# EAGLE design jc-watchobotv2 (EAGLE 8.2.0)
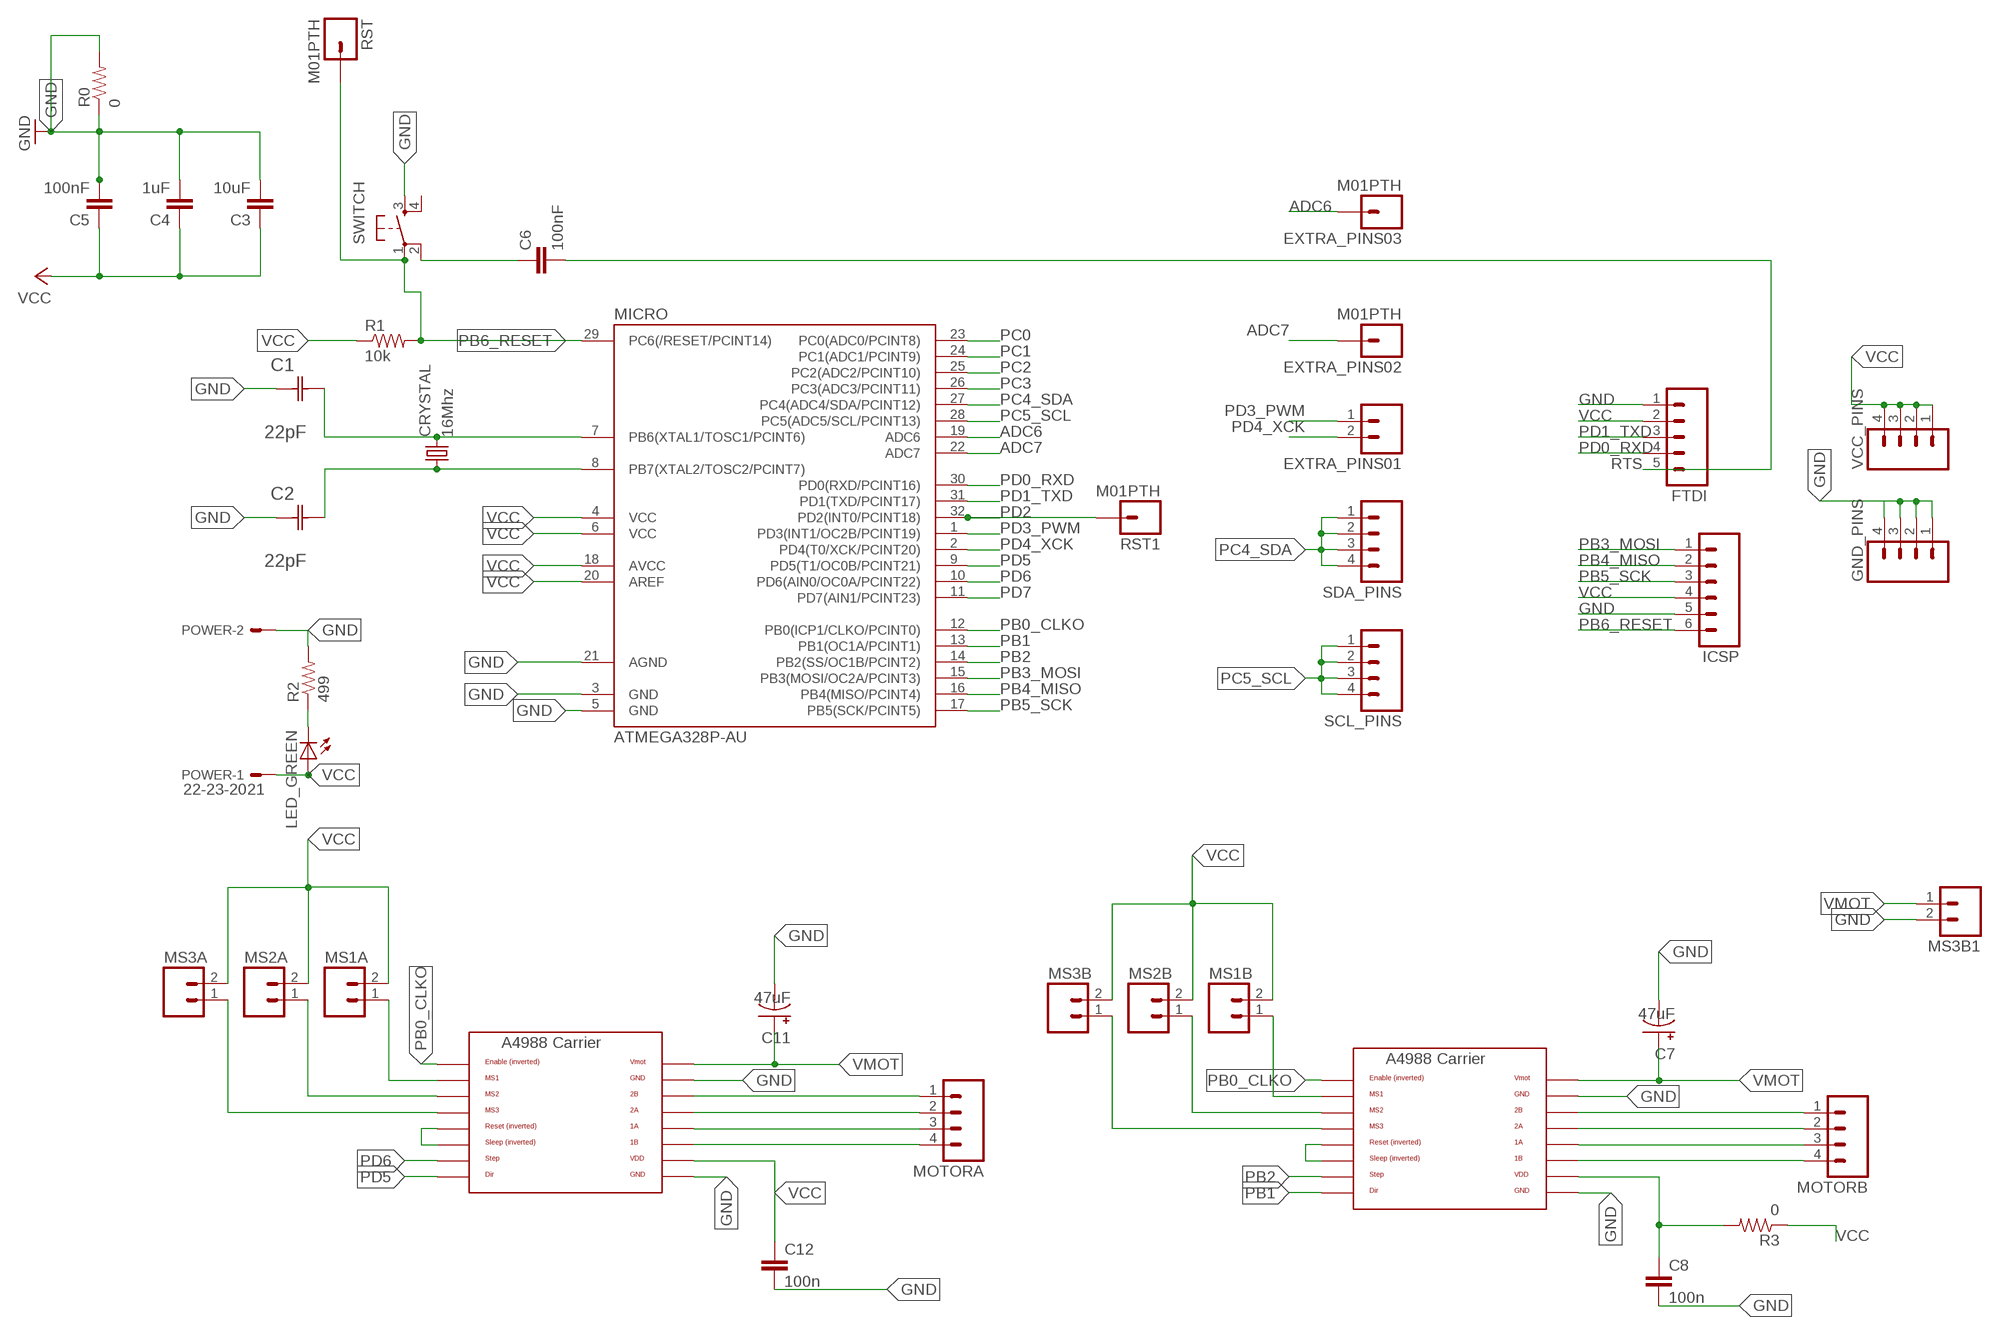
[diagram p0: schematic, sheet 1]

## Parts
C1  22pF  0612ZC225MAT2A  [CAPC3216X178N]
C2  22pF  0612ZC225MAT2A  [CAPC3216X178N]
C3  10uF  CAP1206  [1206]
C4  1uF  CAP1206  [1206]
C5  100nF  CAP1206  [1206]
C6  100nF  CAP1206  [1206]
C7  47uF  MCGPR50V107M8X11  [MCGPR50V107M8X11]
C8  100n  CAP1206  [1206]
C11  47uF  MCGPR50V107M8X11  [MCGPR50V107M8X11]
C12  100n  CAP1206  [1206]
CRYSTAL  16Mhz  CSM-7X-DU  [CSM-7X-DU]
EXTRA_PINS01  M02  [02P]
EXTRA_PINS02  M01PTH  [1X01]
EXTRA_PINS03  M01PTH  [1X01]
FTDI  M05  [05P]
GND_PINS  M04  [04P]
ICSP  M06  [06P]
LED_GREEN  LED1206  [1206]
MICRO  ATMEGA328P-AU  ATMEGA48/88/168-AU  [TQFP32-08]
MOTORA  M04  [04P]
MOTORA_CARRIER  A4988BREAKOUT  [A4988BREAKOUT]
MOTORB  M04  [04P]
MOTORB_CARRIER  A4988BREAKOUT  [A4988BREAKOUT]
MS1A  M02  [02P]
MS1B  M02  [02P]
MS2A  M02  [02P]
MS2B  M02  [02P]
MS3A  M02  [02P]
MS3B  M02  [02P]
MS3B1  M02  [02P]
POWER  22-23-2021  [22-23-2021]
R0  0  RESISTOR1206  [1206]
R1  10k  RESISTOR1206  [1206]
R2  499  RESISTOR1206  [1206]
R3  0  RESISTOR1206  [1206]
RST  M01PTH  [1X01]
RST1  M01PTH  [1X01]
SCL_PINS  M04  [04P]
SDA_PINS  M04  [04P]
SWITCH  6MM_SWITCH6MM_SWITCH  [6MM_SWITCH]
VCC_PINS  M04  [04P]

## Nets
ADC6: EXTRA_PINS03.1 MICRO.19(ADC6)
ADC7: EXTRA_PINS02.1 MICRO.22(ADC7)
GND: C1.1(C1) C2.1(C1) C3.2 C4.2 C5.2 C7.- C8.2 C11.- C12.2 FTDI.1 GND_PINS.1 GND_PINS.2 GND_PINS.3 GND_PINS.4 ICSP.5 MICRO.3(GND) MICRO.5(GND) MICRO.21(AGND) MOTORA_CARRIER.GND MOTORA_CARRIER.GND@0(GND) MOTORB_CARRIER.GND MOTORB_CARRIER.GND@0(GND) MS3B1.2 POWER.2 R0.1 R0.2 R2.2 SWITCH.3(S)
N$1: MOTORB_CARRIER.MS1 MS1B.1
N$3: MOTORA_CARRIER.MS1 MS1A.1
N$4: MOTORA_CARRIER.MS2 MS2A.1
N$5: MOTORA_CARRIER.MS3 MS3A.1
N$6: MOTORA_CARRIER.RST MOTORA_CARRIER.SLP(SLEEP)
N$7: MOTORB_CARRIER.MS2 MS2B.1
N$8: MOTORB_CARRIER.MS3 MS3B.1
N$9: MOTORB_CARRIER.RST MOTORB_CARRIER.SLP(SLEEP)
N$11: MOTORA.1 MOTORA_CARRIER.2B
N$12: MOTORA.2 MOTORA_CARRIER.2A
N$13: MOTORA.3 MOTORA_CARRIER.1A
N$14: MOTORA.4 MOTORA_CARRIER.1B
N$16: MOTORB.1 MOTORB_CARRIER.2B
N$17: MOTORB.2 MOTORB_CARRIER.2A
N$18: MOTORB.3 MOTORB_CARRIER.1A
N$19: MOTORB.4 MOTORB_CARRIER.1B
N$22: C6.1 SWITCH.2(P1)
N$26: LED_GREEN.2(C) R2.1
PB0_CLKO: MICRO.12(PB0(ICP1/CLKO/PCINT0)) MOTORA_CARRIER.EN MOTORB_CARRIER.EN
PB1: MICRO.13(PB1(OC1A/PCINT1)) MOTORB_CARRIER.DIR
PB2: MICRO.14(PB2(SS/OC1B/PCINT2)) MOTORB_CARRIER.STEP
PB3_MOSI: ICSP.1 MICRO.15(PB3(MOSI/OC2A/PCINT3))
PB4_MISO: ICSP.2 MICRO.16(PB4(MISO/PCINT4))
PB5_SCK: ICSP.3 MICRO.17(PB5(SCK/PCINT5))
PB6_RESET: ICSP.6 MICRO.29(PC6(/RESET/PCINT14)) R1.2 RST.1 SWITCH.1(P)
PB6_XTAL1: C1.2(C2) CRYSTAL.2 MICRO.7(PB6(XTAL1/TOSC1/PCINT6))
PB7_XTAL2: C2.2(C2) CRYSTAL.1 MICRO.8(PB7(XTAL2/TOSC2/PCINT7))
PC0: MICRO.23(PC0(ADC0/PCINT8))
PC1: MICRO.24(PC1(ADC1/PCINT9))
PC2: MICRO.25(PC2(ADC2/PCINT10))
PC3: MICRO.26(PC3(ADC3/PCINT11))
PC4_SDA: MICRO.27(PC4(ADC4/SDA/PCINT12)) SDA_PINS.1 SDA_PINS.2 SDA_PINS.3 SDA_PINS.4
PC5_SCL: MICRO.28(PC5(ADC5/SCL/PCINT13)) SCL_PINS.1 SCL_PINS.2 SCL_PINS.3 SCL_PINS.4
PD0_RXD: FTDI.4 MICRO.30(PD0(RXD/PCINT16))
PD1_TXD: FTDI.3 MICRO.31(PD1(TXD/PCINT17))
PD2: MICRO.32(PD2(INT0/PCINT18)) RST1.1
PD3_PWM: EXTRA_PINS01.1 MICRO.1(PD3(INT1/OC2B/PCINT19))
PD4_XCK: EXTRA_PINS01.2 MICRO.2(PD4(T0/XCK/PCINT20))
PD5: MICRO.9(PD5(T1/OC0B/PCINT21)) MOTORA_CARRIER.DIR
PD6: MICRO.10(PD6(AIN0/OC0A/PCINT22)) MOTORA_CARRIER.STEP
PD7: MICRO.11(PD7(AIN1/PCINT23))
RTS: C6.2 FTDI.5
VCC: C3.1 C4.1 C5.1 C8.1 C12.1 FTDI.2 ICSP.4 LED_GREEN.1(A) MICRO.4(VCC) MICRO.6(VCC) MICRO.18(AVCC) MICRO.20(AREF) MOTORA_CARRIER.VDD MOTORB_CARRIER.VDD MS1A.2 MS1B.2 MS2A.2 MS2B.2 MS3A.2 MS3B.2 POWER.1 R1.1 R3.1 R3.2 VCC_PINS.1 VCC_PINS.2 VCC_PINS.3 VCC_PINS.4
VMOT: C7.+ C11.+ MOTORA_CARRIER.VMOT MOTORB_CARRIER.VMOT MS3B1.1
Unconnected: SWITCH.4(S1)

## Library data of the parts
C1 C2 = AVX_By_element14_Batch_1:0612ZC225MAT2A: Capacitor 1206; MPN: 0612ZC225MAT2A; OC_FARNELL: -; OC_NEWARK: 12N3209; SUPPLIER: AVX; TOLERANCE: ±20%; VALUE: 2.2µF; VOLTAGERATING: 10V
C3-C6 C8 C12 = 01_SparkFun:CAP: Capacitor
C7 C11 = Ryan:MCGPR50V107M8X11
CRYSTAL = 01_FAB_Hello:CSM-7X-DU: SMD CRYSTAL; OC_FARNELL: unknown; OC_NEWARK: unknown
EXTRA_PINS01 MS1A MS1B MS2A MS2B MS3A MS3B MS3B1 = con-amp-quick:M02: AMP QUICK CONNECTOR; OC_FARNELL: unknown; OC_NEWARK: unknown
EXTRA_PINS02 EXTRA_PINS03 RST RST1 = 01_SparkFun:M01: Header 1
FTDI = con-amp-quick:M05: AMP QUICK CONNECTOR; OC_FARNELL: unknown; OC_NEWARK: unknown
GND_PINS MOTORA MOTORB SCL_PINS SDA_PINS VCC_PINS = con-amp-quick:M04: AMP QUICK CONNECTOR; OC_FARNELL: unknown; OC_NEWARK: unknown
ICSP = con-amp-quick:M06: AMP QUICK CONNECTOR; OC_FARNELL: unknown; OC_NEWARK: unknown
LED_GREEN = 01_FAB_Hello:LED
MICRO = atmega8:ATMEGA48/88/168
MOTORA_CARRIER MOTORB_CARRIER = RepRapjr:A4988BREAKOUT
POWER = con-molex:22-23-2021: .100" (2.54mm) Center Header - 2 Pin; MF: MOLEX; MPN: 22-23-2021; OC_FARNELL: 1462926; OC_NEWARK: 25C3832
R0 R1-R3 = 01_SparkFun:RESISTOR: Resistor
SWITCH = 01_FAB_Hello:6MM_SWITCH: OMRON SWITCH

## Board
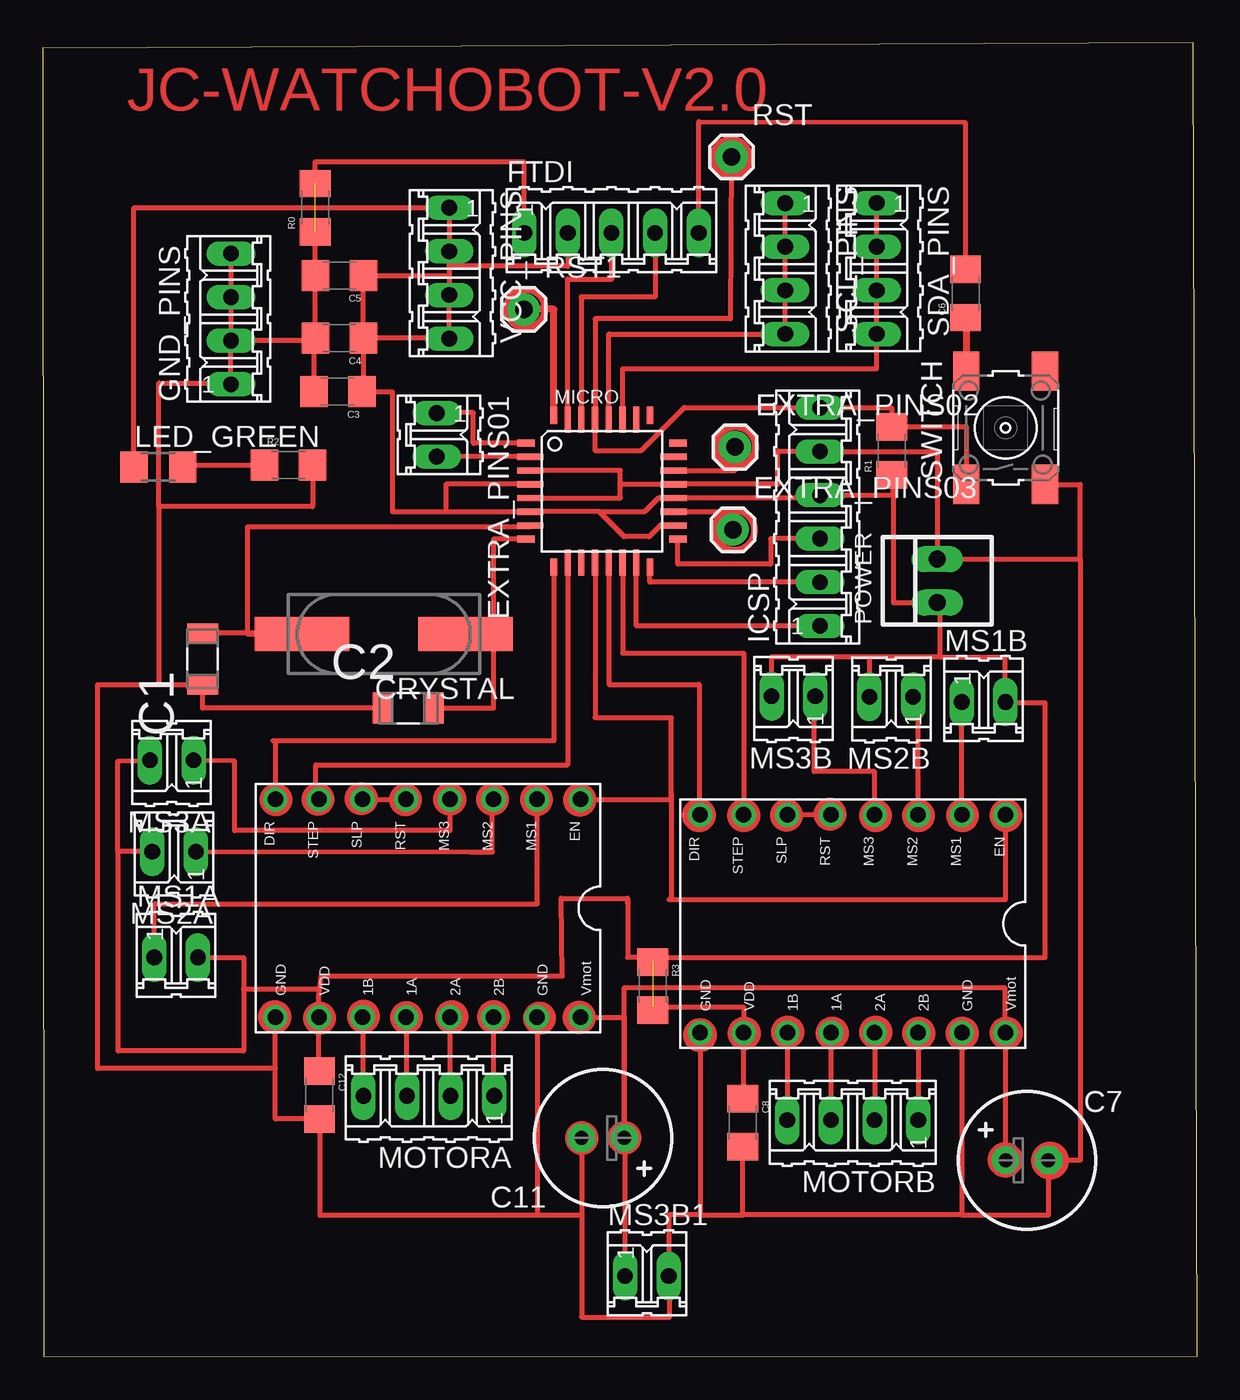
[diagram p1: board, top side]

Size 67.2 x 76.52 mm. Coordinates in mm from the lower left corner, seen from the top.
Outline: 0.03,0 67.2,0.02 66.99,76.52 0,76.22 0.03,0
Copper layers (1*16): Top 0.035mm / dielectric 1.5mm / Bottom 0.035mm
Design rules "default *": minimum track width 10mil, minimum drill 24mil, track to track 8mil, track to pad 8mil, pad to pad 8mil, via to via 8mil, smd to smd 8mil, copper to edge 40mil, drill to drill 8mil, minimum pad ring 10mil, minimum via ring 8mil, stop-mask expansion 4mil, vias tented up to drill 0mil, thermal gap 10mil

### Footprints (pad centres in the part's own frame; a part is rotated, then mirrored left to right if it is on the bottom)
CAPC3216X178N = smd 1.118 x 1.803: 1 -1.499,0; 2 1.499,0
1206 = smd 1.6 x 1.8: 1 -1.4,0; 2 1.4,0
MCGPR50V107M8X11 = drill 0.813 pad 1.6: + -1.25,0 | drill 0.813 pad 1.6 octagon: - 1.25,0
CSM-7X-DU = smd 5.5 x 2: 1 -4.75,0; 2 4.75,0
02P = drill 0.914 long: 1 -1.27,0; 2 1.27,0
1X01 = drill 1.016 pad 1.88: 1 0,0
05P = drill 0.914 long: 1 -5.08,0; 2 -2.54,0; 3 0,0; 4 2.54,0; 5 5.08,0
04P = drill 0.914 long: 1 -3.81,0; 2 -1.27,0; 3 1.27,0; 4 3.81,0
06P = drill 0.914 long: 1 -6.35,0; 2 -3.81,0; 3 -1.27,0; 4 1.27,0; 5 3.81,0; 6 6.35,0
1206' = smd 1.6 x 1.803: 1 -1.422,0; 2 1.422,0
TQFP32-08 = smd 1.016 x 0.406: 1 -4.42,2.8; 8 -4.42,-2.8; 17 4.42,-2.8; 24 4.42,2.8 | smd 1.524 x 0.356: 2 -4.166,2; 3 -4.166,1.2; 4 -4.166,0.4; 5 -4.166,-0.4; 6 -4.166,-1.2; 7 -4.166,-2; 18 4.166,-2; 19 4.166,-1.2; 20 4.166,-0.4; 21 4.166,0.4; 22 4.166,1.2; 23 4.166,2 | smd 0.406 x 1.016: 9 -2.8,-4.42; 16 2.8,-4.42; 25 2.8,4.42; 32 -2.8,4.42 | smd 0.356 x 1.524: 10 -2,-4.166; 11 -1.2,-4.166; 12 -0.4,-4.166; 13 0.4,-4.166; 14 1.2,-4.166; 15 2,-4.166; 26 2,4.166; 27 1.2,4.166; 28 0.4,4.166; 29 -0.4,4.166; 30 -1.2,4.166; 31 -2,4.166
A4988BREAKOUT = drill 0.9: 1A 8.89,1.27; 1B 11.43,1.27; 2A 6.35,1.27; 2B 3.81,1.27; DIR 16.51,-11.43; EN -1.27,-11.43; GND 16.51,1.27; GND@0 1.27,1.27; MS1 1.27,-11.43; MS2 3.81,-11.43; MS3 6.35,-11.43; RST 8.89,-11.43; SLP 11.43,-11.43; STEP 13.97,-11.43; VDD 13.97,1.27; VMOT -1.27,1.27
22-23-2021 = drill 1 long: 1 -1.27,0; 2 1.27,0
6MM_SWITCH = smd 2.286 x 1.524: 1 -3.302,2.286; 2 3.302,2.286; 3 -3.302,-2.286; 4 3.302,-2.286

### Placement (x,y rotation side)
C1  9.3,40.63 90 top
C2  21.27,37.78 0 top
C3  17.17,56.2 180 top
C4  17.26,59.32 180 top
C5  17.26,62.96 180 top
C6  53.72,61.92 90 top
C7  57.3,11.43 0 top
C8  40.76,13.63 270 top
C11  32.61,12.73 180 top
C12  16.1,15.23 270 top
CRYSTAL  19.85,42.09 180 top
EXTRA_PINS01  22.93,53.69 270 top
EXTRA_PINS02  40.3,52.98 0 top
EXTRA_PINS03  40.17,48.17 0 top
FTDI  33.1,65.44 0 top
GND_PINS  10.94,60.44 90 top
ICSP  45.25,48.91 90 top
LED_GREEN  [1206']  6.72,51.82 0 top
MICRO  32.55,50.41 0 top
MOTORA  22.47,15.19 180 top
MOTORA_CARRIER  30.04,21.03 180 top
MOTORB  47.15,13.78 180 top
MOTORB_CARRIER  54.77,20.13 180 top
MS1A  7.76,23.25 0 top
MS1B  54.77,38.13 0 top
MS2A  7.64,29.41 180 top
MS2B  49.4,38.44 180 top
MS3A  7.5,34.73 180 top
MS3B  43.7,38.45 180 top
MS3B1  35.17,4.69 0 top
POWER  52.07,45.18 90 top
R0  15.85,66.92 90 top
R1  49.42,52.76 90 top
R2  14.3,51.92 0 top
R3  35.51,21.58 270 top
RST  40.09,69.88 0 top
RST1  28,61 0 top
SCL_PINS  43.22,63.37 270 top
SDA_PINS  48.55,63.38 270 top
SWITCH  56.06,54.1 90 top
VCC_PINS  23.66,63.11 270 top

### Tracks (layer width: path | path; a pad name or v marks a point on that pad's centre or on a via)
ADC6
  Top 0.305: MICRO.19 40.17,49.21 EXTRA_PINS03.1
ADC7
  Top 0.305: MICRO.22 40.3,51.61 EXTRA_PINS02.1
GND  (1 unrouted)
  Top 0.305: 28.38,51.6 MICRO.3 | C2.1 9.3,37.78 C1.1 6.75,39.14 | 38.24,18.86 MOTORB_CARRIER.GND 38.26,8.25 | C4.2 15.86,59.17 GND_PINS.2 | C4.2 C5.2 15.86,65.52 R0.1 | GND_PINS.4 GND_PINS.3 GND_PINS.2 | GND_PINS.2 GND_PINS.1 10.94,56.71 6.75,56.71 6.75,49.51 | 6.75,49.51 6.75,39.14 | 38.26,8.25 40.76,8.25 | 16.12,8.25 16.12,13.83 C12.2 13.53,13.83 13.53,16.78 | MOTORA_CARRIER.GND@0 28.77,8.25 | C11.- 31.36,8.25 | 53.51,8.25 58.55,8.25 C7.- 60.4,11.44 60.4,46.45 | 53.51,8.25 40.76,8.25 | MOTORB_CARRIER.GND@0 53.51,8.25 | 13.53,16.78 MOTORA_CARRIER.GND | SWITCH.3 60.4,50.8 60.4,46.45 | 60.4,46.45 POWER.2 52.07,52.72 ICSP.5 45.25,52.75 42.79,52.75 42.79,50.81 MICRO.21 33.62,50.81 | C4.2 15.77,59.32 C3.2 | R2.2 15.7,49.51 6.75,49.51 | R0.2 15.85,69.59 28.01,69.59 FTDI.1 | 16.12,8.22 16.12,8.25 | 16.12,8.25 28.77,8.25 | 28.77,8.25 31.36,8.25 | 31.36,8.25 31.36,2.29 36.5,2.29 36.5,4.69 MS3B1.2 36.44,8.25 38.26,8.25 | 40.76,8.25 C8.2 | 6.75,39.14 6.75,39.13 3.19,39.13 3.19,16.78 13.53,16.78 | 33.62,50.81 33.62,51.61 MICRO.3 | MICRO.3 | MICRO.5 33.62,50.01 33.62,50.81
N$1
  Top 0.305: MOTORB_CARRIER.MS1 MS1B.1 | MS1B.1
N$3
  Top 0.305: MS1A.1 6.49,26.37 28.78,26.37 MOTORA_CARRIER.MS1
N$4
  Top 0.305: MS2A.1 24.9,29.39 26.18,29.39 26.18,32.46 MOTORA_CARRIER.MS2
N$5
  Top 0.305: 23.68,32.46 MOTORA_CARRIER.MS3 23.69,30.64 11.16,30.64 11.16,34.69 MS3A.1
N$6
  Top 0.305: MOTORA_CARRIER.SLP MOTORA_CARRIER.RST
N$7
  Top 0.305: MOTORB_CARRIER.MS2 50.96,38.44 MS2B.1
N$8
  Top 0.305: MOTORB_CARRIER.MS3 48.43,34.07 44.9,34.07 44.9,38.45 MS3B.1
N$9
  Top 0.305: MOTORB_CARRIER.RST MOTORB_CARRIER.SLP
N$11
  Top 0.305: MOTORA_CARRIER.2B 26.23,15.19 MOTORA.1
N$12
  Top 0.305: MOTORA_CARRIER.2A 23.69,15.19 MOTORA.2
N$13
  Top 0.305: MOTORA_CARRIER.1A 21.15,15.19 MOTORA.3
N$14
  Top 0.305: MOTORA_CARRIER.1B 18.61,15.19 MOTORA.4
N$16
  Top 0.305: MOTORB_CARRIER.2B MOTORB.1
N$17
  Top 0.305: MOTORB_CARRIER.2A MOTORB.2
N$18
  Top 0.305: MOTORB_CARRIER.1A MOTORB.3
N$19
  Top 0.305: MOTORB_CARRIER.1B MOTORB.4
N$22
  Top 0.406: C6.1 53.77,60.52 SWITCH.2
N$26
  Top 0.305: LED_GREEN.2 8.14,51.92 R2.1
PB0_CLKO
  Top 0.305: MOTORB_CARRIER.EN 56.04,26.62 36.45,26.62 36.59,26.62 36.59,32.78 | MICRO.12 32.15,37.22 36.59,37.22 36.59,32.78 | MOTORA_CARRIER.EN 36.59,32.46 36.59,32.78
PB1
  Top 0.305: MICRO.13 32.95,39.15 38.2,39.15 38.2,31.56 MOTORB_CARRIER.DIR
PB2
  Top 0.305: MICRO.14 33.75,40.97 40.79,40.97 40.79,31.56 MOTORB_CARRIER.STEP
PB3_MOSI
  Top 0.305: ICSP.1 34.55,42.56 MICRO.15
PB4_MISO
  Top 0.305: ICSP.2 35.35,45.1 MICRO.16
PB5_SCK
  Top 0.305: 36.97,47.64 MICRO.17 36.97,46.15 42.38,46.15 42.38,47.64 ICSP.3
PB6_RESET
  Top 0.305: RST.1 40.03,60.45 32.15,60.45 MICRO.29 32.15,52.77 34.84,52.77 37.35,55.28 37.36,55.26 ICSP.6 49.42,55.26 R1.2 53.77,54.16 SWITCH.1
PB6_XTAL1
  Top 0.305: MICRO.7 28.38,48.33 11.91,48.33 11.91,42.09 CRYSTAL.2 15.1,42.13 C1.2
PB7_XTAL2
  Top 0.305: MICRO.8 26.25,47.61 26.25,42.07 | 26.25,42.07 24.6,42.07 CRYSTAL.1 | C2.2 26.25,37.78 26.25,42.07
PC4_SDA
  Top 0.305: SDA_PINS.1 SDA_PINS.2 SDA_PINS.3 SDA_PINS.4 48.55,57.54 33.75,57.54 MICRO.27
PC5_SCL
  Top 0.305: SCL_PINS.1 SCL_PINS.2 SCL_PINS.3 SCL_PINS.4 32.95,59.56 MICRO.28
PD0_RXD
  Top 0.305: FTDI.4 35.64,61.72 31.34,61.72 31.34,54.57 MICRO.30
PD1_TXD
  Top 0.305: MICRO.31 30.55,62.76 33.13,62.76 33.13,65.44 FTDI.3
PD2
  Top 0.406: MICRO.32 29.75,61 RST1.1
PD3_PWM
  Top 0.305: MICRO.1 25.06,53.21 25.06,54.97 22.93,54.97 EXTRA_PINS01.1
PD4_XCK
  Top 0.305: MICRO.2 EXTRA_PINS01.2
PD5
  Top 0.305: MICRO.9 29.75,35.87 13.4,35.87 13.53,35.87 MOTORA_CARRIER.DIR
PD6
  Top 0.305: MICRO.10 30.55,34.47 15.89,34.47 15.89,32.46 MOTORA_CARRIER.STEP
RTS
  Top 0.305: FTDI.5 38.2,71.93 53.7,71.89 53.7,63.32 C6.2
VCC  (1 unrouted)
  Top 0.305: C4.1 23.66,59.32 VCC_PINS.4 VCC_PINS.3 23.66,62.96 | 23.66,63.51 VCC_PINS.2 VCC_PINS.1 5.3,66.92 LED_GREEN.1 | 23.66,63.51 23.66,62.96 | C4.1 C5.1 23.66,62.96 | C4.1 18.83,59.32 | 28.38,49.18 MICRO.6 | 23.46,49.21 MICRO.6 | 23.46,49.21 20.35,49.21 20.35,56.2 C3.1 18.66,56.2 C4.1 | MICRO.4 23.46,50.81 23.46,49.21 | MS3B.2 42.43,40.76 48.11,40.76 | 48.11,40.76 48.11,38.44 | 52.23,40.76 56.04,40.76 MS1B.2 56.04,38.08 58.36,38.08 58.36,23.25 35.51,23.25 | 52.23,40.76 48.11,40.76 | 34.05,26.4 34.05,26.7 | 34.05,26.4 34.05,23.25 35.51,23.25 | 52.23,40.76 52.23,43.91 POWER.1 49.51,43.91 49.51,50.18 | 36.71,48.46 MICRO.18 35.94,48.41 35.29,47.76 33.84,47.76 32.39,49.21 | 32.39,49.21 35.04,49.21 35.84,50.01 MICRO.20 45.25,50.01 ICSP.4 49.51,50.18 | 32.39,49.21 MICRO.6 | R1.1 49.51,51.36 49.51,50.18 | FTDI.2 30.56,63.51 23.66,63.51 | C8.1 40.8,15.03 MOTORB_CARRIER.VDD 40.8,20.36 35.51,20.36 R3.2 | C12.1 16.07,16.63 MOTORA_CARRIER.VDD 16.07,21.11 16.1,21.41 | R3.1 35.51,23.25 | 16.1,21.41 16.18,22.15 30.24,22.15 30.17,26.7 34.05,26.7 | MS3A.2 4.37,34.69 4.37,29.41 | 11.68,21.41 16.1,21.41 | 11.68,21.41 11.68,17.8 4.37,17.8 4.37,29.41 | MS2A.2 4.37,29.41 | MS1A.2 11.68,23.25 11.68,21.41 | 34.05,26.7 34.05,26.4
  Top 0.406: 48.11,38.44 MS2B.2
VMOT
  Top 0.305: MOTORA_CARRIER.VMOT 33.86,19.76 C11.+ | C7.+ MOTORB_CARRIER.VMOT 56,18.86 56,21.5 33.86,21.5 C11.+ | MS3B1.1 33.9,12.73 C11.+
(copper drawn outside any net)
  shapes: Top circle x40

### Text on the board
Top: JC-WATCHOBOT-V2.0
